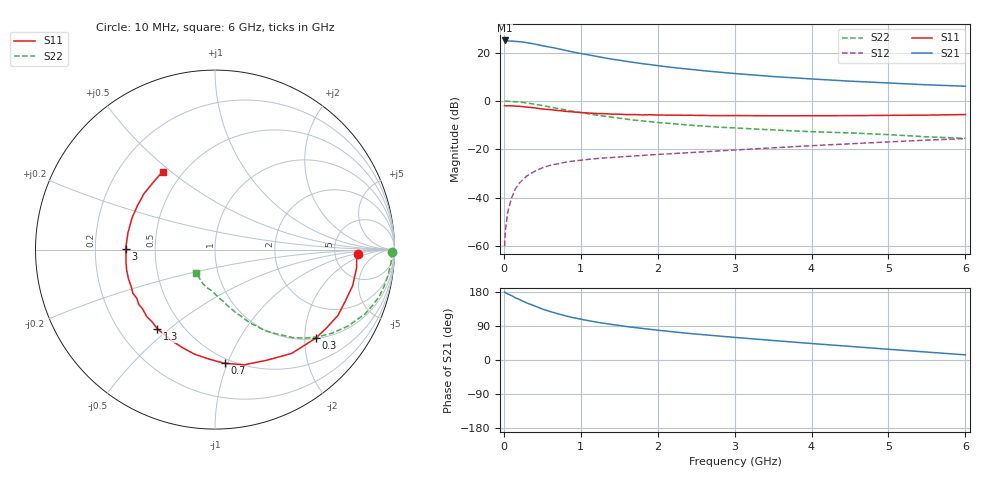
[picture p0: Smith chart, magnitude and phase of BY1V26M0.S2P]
! SIEMENS Small Signal Semiconductors
! BFY420
! Si NPN RF SIEGET Grounded Emitter Transistor in MICRO-X
! VCE = 1.25 V  IC = 6 mA
! Common Emitter S-Parameters:  October  1996
# GHz  S  MA  R  50
!  f  S11  S21  S12  S22
! GHz  MAG  ANG  MAG  ANG  MAG  ANG  MAG  ANG
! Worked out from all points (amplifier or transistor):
!   36 points, 10 MHz to 6 GHz, reference 50 ohm
!   highest |S21| = 25.0 dB at 10 MHz (marker M1)
!   |S21| within 3 dB of that: start of sweep to 641.2 MHz
!   unconditionally stable (mu >= 1): 2.902 GHz to end of sweep
!   at 250 MHz: K = 0.12, MSG = 28.4 dB, |S12| = -32.4 dB
!   at 1.4 GHz: K = 0.60, MSG = 20.3 dB, |S12| = -23.4 dB
!   at 6 GHz: K = 1.15, MAG = 8.5 dB, |S12| = -15.6 dB
!   S11 on the Smith chart (normalised r, x): 10 MHz: 8.78, -1.22; 300 MHz: 1.01, -2.26; 700 MHz: 0.46, -0.98; 1.3 GHz: 0.36, -0.45; 3 GHz: 0.34, +0.00; 6 GHz: 0.39, +0.47
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0.01  0.7991 -1.8  17.75 179.8  0.001 107.3  0.9872 -0.8
0.02  0.7902 -2.9  17.66 177.5  0.0021 92.1  0.9843 -1.6
0.05  0.7954 -7.3  17.34 174.3  0.005 90.4  0.9839 -4.0
0.1  0.7928 -14.6  17.27 170.1  0.0098 81.2  0.9752 -8.1
0.15  0.7811 -21.2  17 164.1  0.0152 78.4  0.9646 -12.1
0.2  0.7771 -28.1  16.75 160.1  0.02 76.3  0.9517 -15.9
0.3  0.7472 -41.4  15.99 150.4  0.0283 69.6  0.9086 -23.3
0.4  0.7188 -53.6  14.99 142.7  0.0351 63.9  0.8557 -29.8
0.5  0.6804 -65.0  13.82 134.5  0.0415 59.0  0.8028 -35.4
0.6  0.6621 -75.7  12.96 128.1  0.0467 54.7  0.7504 -40.4
0.7  0.636 -85.1  12.03 122.1  0.0502 51.4  0.7001 -44.8
0.8  0.6108 -93.2  11.08 116.6  0.0541 48.3  0.6532 -48.6
0.9  0.5936 -101.1  10.24 111.8  0.0573 46.1  0.6109 -51.5
1.1  0.5626 -115.1  8.96 103.8  0.0623 43.0  0.5429 -57.2
1.3  0.5459 -126.1  7.822 97.0  0.0663 40.3  0.4855 -61.4
1.7  0.5231 -144.3  6.211 85.7  0.0732 38.3  0.3999 -68.4
2.2  0.5089 -161.3  4.897 74.4  0.0818 36.3  0.3386 -75.2
3  0.498 179.5  3.685 59.7  0.0969 34.6  0.2773 -83.8
3.5  0.494 168.9  3.192 51.5  0.1075 33.1  0.2518 -89.0
4.5  0.4968 150.3  2.562 35.9  0.1303 28.1  0.2188 -100.5
5.5  0.5095 132.0  2.154 20.9  0.1552 21.7  0.1813 -118.2
6  0.5234 123.8  2.012 13.6  0.1665 17.8  0.1684 -130.0
